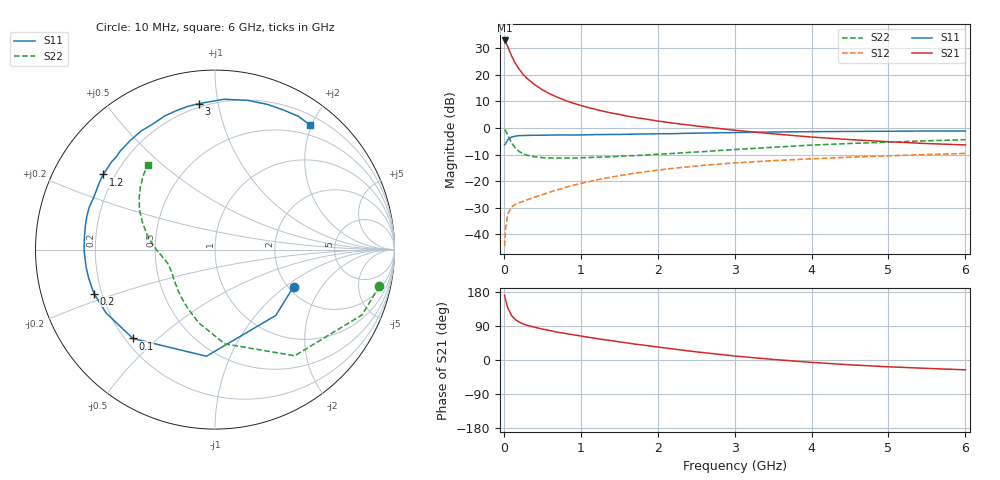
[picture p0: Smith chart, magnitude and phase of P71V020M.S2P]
! SIEMENS Small Signal Semiconductors
! BFP196
! Si NPN RF Bipolar Junction Transistor in SOT143
! VCE = 1 V  IC = 20 mA
! Common Emitter S-Parameters:  May  1996
# GHz  S  MA  R  50
!  f  S11  S21  S12  S22
! GHz  MAG  ANG  MAG  ANG  MAG  ANG  MAG  ANG
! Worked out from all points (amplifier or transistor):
!   36 points, 10 MHz to 6 GHz, reference 50 ohm
!   highest |S21| = 32.9 dB at 10 MHz (marker M1)
!   |S21| within 3 dB of that: start of sweep to 60.78 MHz
!   unconditionally stable (mu >= 1): 632.5 MHz to 5.185 GHz; 5.776 GHz to end of sweep
!   at 250 MHz: K = 0.62, MSG = 23.9 dB, |S12| = -27.6 dB
!   at 1.4 GHz: K = 1.12, MAG = 9.9 dB, |S12| = -18.5 dB
!   at 6 GHz: K = 1.01, MAG = 1.1 dB, |S12| = -9.6 dB
!   S11 on the Smith chart (normalised r, x): 10 MHz: 2.14, -1.15; 100 MHz: 0.23, -0.42; 200 MHz: 0.17, -0.17; 1.2 GHz: 0.16, +0.30; 3 GHz: 0.18, +0.88; 6 GHz: 0.34, +1.98
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0.01  0.4841 -25.2  44.1 170.7  0.006 80.0  0.9381 -12.5
0.02  0.4993 -47.3  41.84 160.4  0.0118 72.0  0.8967 -23.9
0.05  0.596 -94.6  34.07 138.2  0.0237 53.9  0.7398 -53.1
0.1  0.6739 -132.7  22.72 117.4  0.0327 41.8  0.5278 -84.1
0.15  0.702 -149.7  16.32 106.6  0.0367 37.3  0.4183 -102.4
0.2  0.7173 -160.0  12.65 99.8  0.0392 37.8  0.3601 -115.1
0.25  0.7212 -166.9  10.19 95.1  0.0417 38.7  0.3262 -124.9
0.3  0.7248 -172.0  8.578 91.7  0.0444 40.3  0.308 -131.6
0.4  0.7295 -179.7  6.515 86.3  0.0499 43.4  0.2862 -141.9
0.5  0.7305 175.2  5.213 81.8  0.0555 46.2  0.2763 -148.6
0.6  0.7342 169.9  4.359 77.5  0.0625 48.5  0.272 -153.2
0.7  0.7377 165.3  3.758 73.3  0.0688 49.8  0.2714 -156.7
0.9  0.7358 157.5  2.928 66.7  0.0836 51.3  0.2721 -162.1
1.1  0.7447 149.9  2.413 60.0  0.0977 51.3  0.2786 -165.6
1.2  0.7509 146.1  2.22 56.8  0.105 51.1  0.2817 -167.3
1.7  0.7653 130.2  1.578 42.0  0.1408 47.2  0.3024 -174.5
2.2  0.7808 116.4  1.232 29.1  0.1741 41.5  0.3315 179.0
3  0.8182 96.4  0.907 10.6  0.2201 31.1  0.3917 166.7
3.5  0.8393 86.5  0.775 1.5  0.243 24.7  0.4336 159.1
4.5  0.8602 70.1  0.604 -12.7  0.2824 13.2  0.5109 145.8
5.5  0.8758 58.1  0.509 -22.1  0.3168 2.5  0.574 134.3
6  0.8736 52.5  0.48 -25.9  0.3324 -3.3  0.6019 128.6
